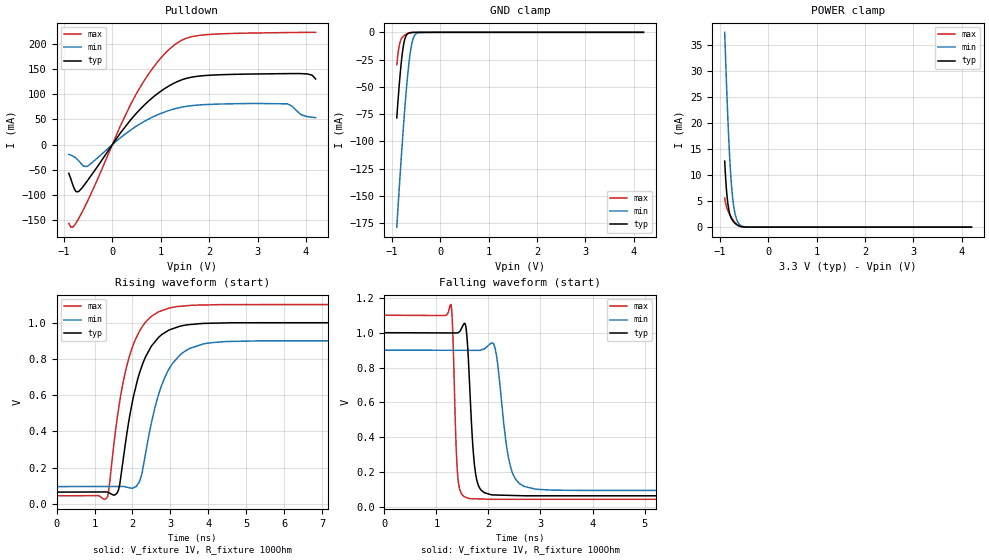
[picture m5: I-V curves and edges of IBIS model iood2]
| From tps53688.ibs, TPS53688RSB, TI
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|   iood2 Model
[Model]   iood2
Model_type   I/O_open_drain
Polarity   Non-Inverting
Enable   Active-Low
Vinl = 0.5
Vinh = 0.6
Vmeas = 0.5
Vref = 1
Cref = 2pF
Rref = 100
|   typ   min   max
C_comp   2.464pF   2.430pF   2.487pF
[Voltage Range]   3.3   2.95   3.6
[Temperature Range]   25   125   -40
[Pullup Reference]   3.3   2.95   3.6
[Pulldown Reference]   0   0   0
[Power Clamp Reference]   3.3   2.95   3.6
[GND Clamp Reference]   0   0   0
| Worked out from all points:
|   slope of the pulldown table from 0 to 0.495 V, typ, clamps not added: 7.97 ohm
|   GND clamp passes 1 mA (typ) near -0.66 V on its own axis
|   POWER clamp passes 1 mA (typ) near -0.71 V on its own axis
|   falling waveform, V_fixture 1V, R_fixture 100Ohm: 20-80 % time 108ps typ, 197ps min, 66.2ps max; typ from 1 V to 0.065 V
|   rising waveform, V_fixture 1V, R_fixture 100Ohm: 20-80 % time 588ps typ, 622ps min, 570ps max; typ from 0.065 V to 1 V
[Pulldown]
|   Voltage   I(typ)   I(min)   I(max)
-900mV    -57.13mA   -19.7mA    -156.7mA
-818.4mV  -80.08mA   -22.8mA    -164.1mA
-757.2mV  -92.63mA   -26.6mA    -156.5mA
-696mV    -93.13mA   -32.29mA   -146.7mA
-492mV    -68.58mA   -41.61mA   -107.9mA
451.5mV   57.43mA    33.82mA    93.26mA
879.9mV   97.22mA    56.83mA    157.6mA
1.278V    122.2mA    70.79mA    197.6mA
1.839V    136.5mA    78.96mA    217.4mA
3.614V    141mA      80.91mA    222.5mA
3.889V    141mA      59.91mA    222.8mA
4.2V      130.3mA    53.53mA    222.9mA
[GND Clamp]
|   Voltage   I(typ)   I(min)   I(max)
-900mV    -78.44mA   -178.5mA   -29.6mA
-869.4mV  -59.78mA   -157mA     -17.86mA
-838.8mV  -42.87mA   -136mA     -10.2mA
-792.9mV  -22.07mA   -105.7mA   -5.024mA
-747mV    -8.595mA   -77.46mA   -2.915mA
-685.8mV  -1.734mA   -44.5mA    -1.283mA
-624.6mV  -370.1uA   -19.76mA   -425.1uA
-594mV    -177.9uA   -11.46mA   -217.8uA
-563.4mV  -84.73uA   -5.977mA   -103.7uA
-507.3mV  -19.78uA   -1.452mA   -21.5uA
-12.6mV   0A         0A         0A
4.2V      0A         0A         0A
[POWER Clamp]
|   Voltage   I(typ)   I(min)   I(max)
-900mV    12.7mA     37.48mA    5.606mA
-874.5mV  8.596mA    30.59mA    4.331mA
-843.9mV  5.281mA    22.98mA    3.399mA
-803.1mV  2.855mA    14.51mA    2.56mA
-782.7mV  2.165mA    11.14mA    2.208mA
-762.3mV  1.683mA    8.392mA    1.884mA
-726.6mV  1.134mA    4.931mA    1.374mA
-690.9mV  774.3uA    2.8mA      940.4uA
-645mV    445.7uA    1.282mA    507.8uA
-588.9mV  189.2uA    457.3uA    182.6uA
-354.3mV  574.3nA    4.059uA    109.3nA
4.2V      0A         0A         0A
[Ramp]
R_load = 100
|   typ   min   max
dV/dt_r   0.560777/5.88262e-10   0.482429/6.2439e-10   0.632948/5.70162e-10
dV/dt_f   0.560777/1.07733e-10   0.482429/1.96278e-10   0.632948/6.60849e-11
[Falling Waveform]
V_fixture = 1V
V_fixture_min = 0.9V
V_fixture_max = 1.1V
R_fixture = 100Ohm
C_fixture = 0F
|   Time   V(typ)   V(min)   V(max)
0s        1V         900mV      1.1V
1.276ns   998.6mV    899.2mV    1.161V
1.411ns   999.7mV    899.1mV    172.7mV
1.555ns   1.048V     899mV      57.82mV
1.625ns   781.6mV    899mV      50.09mV
1.82ns    115.6mV    898.9mV    47.46mV
2.112ns   70.01mV    926.5mV    45.12mV
2.436ns   67.45mV    218.8mV    45.12mV
2.879ns   65.42mV    104.9mV    45.12mV
18.5ns    65.37mV    95.95mV    45.09mV
[Rising Waveform]
V_fixture = 1V
V_fixture_min = 0.9V
V_fixture_max = 1.1V
R_fixture = 100Ohm
C_fixture = 0F
|   Time   V(typ)   V(min)   V(max)
0s        65.37mV    95.95mV    45.09mV
1.332ns   66.32mV    96.45mV    36mV
1.592ns   59.94mV    96.55mV    465.5mV
1.863ns   403.6mV    92mV       772mV
2.193ns   727.4mV    129.5mV    956.3mV
2.609ns   898.7mV    545.3mV    1.049V
2.973ns   960.3mV    748.1mV    1.081V
3.504ns   989.1mV    857.6mV    1.095V
4.45ns    998.5mV    895.7mV    1.099V
18.5ns    1V         900mV      1.1V
